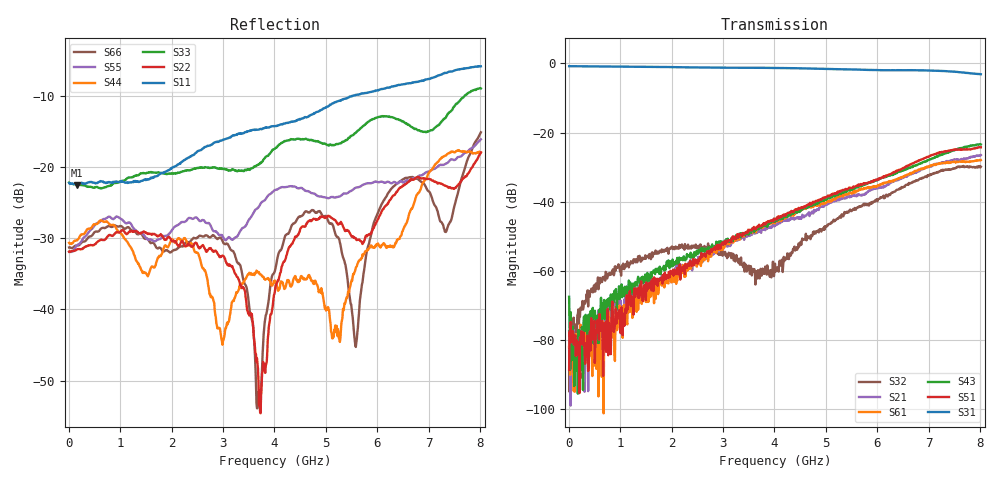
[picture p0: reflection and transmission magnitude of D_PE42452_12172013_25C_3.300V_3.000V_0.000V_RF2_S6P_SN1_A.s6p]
! Device ID: PE42422_06252012
! Dir: z:\David_A\42452\10_28_13_42452_omar_meas\25C\3p300000\RF2
! Serial: 1
! Insertion: A
! Temp: 25C
! VDD: 3.300
! Control_Hi: 3.000
! Control_Lo: 0.000
! Logic State: RF2
! Port 1: RFC
! Port 2: RF1
! Port 3: RF2
! Port 4: RF3
! Port 5: RF4
! Port 6: RF5
! ThroughPath:3-1
! V1 = 0.00
! V2 = 3.00
! V3 = 0.00
! V4 = 0.00
#  Hz  S  RI  R  50
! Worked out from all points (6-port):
!   801 points, 10 MHz to 8.01 GHz, reference 50 ohm
!   strongest paths, dB at 10 MHz, 2.01 GHz, 4.01 GHz, 6.01 GHz, 8.01 GHz:
!     S31: -0.8, -1.1, -1.3, -1.9, -3.1
!     S51: -88.6, -60.6, -45.2, -33.5, -24.3
!     S43: -67.5, -57.6, -45.6, -33.6, -23.4
!     S61: -82.1, -62.0, -46.3, -35.2, -28.0
!     S21: -77.4, -61.4, -46.9, -36.0, -26.5
!     S32: -82.0, -52.9, -57.9, -39.3, -29.9
!   lowest |S11| = -22.5 dB at 160 MHz (marker M1), VSWR 1.16, Z = 57.7 - j2.21 ohm
!   |S11| at or under -10 dB: start of sweep to 5.524 GHz
